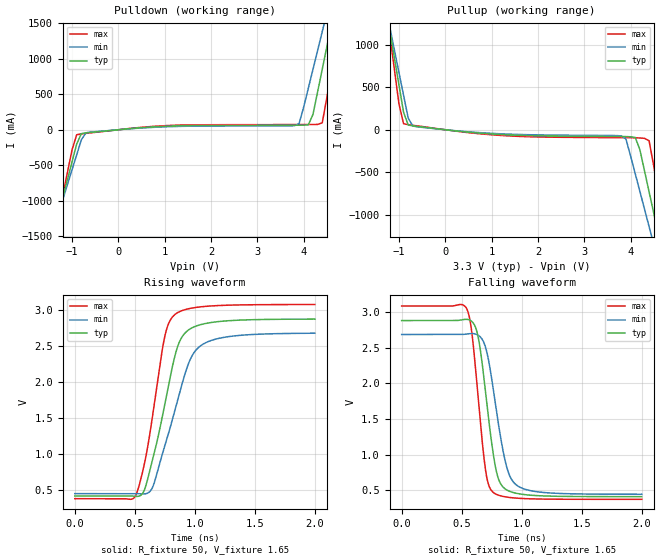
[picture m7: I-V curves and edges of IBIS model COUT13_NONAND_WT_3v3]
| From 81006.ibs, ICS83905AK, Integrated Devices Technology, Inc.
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[Model] COUT13_NONAND_WT_3v3
Model_type   Output
Polarity   Non-Inverting
|   typ   min   max
C_comp   2pF   1.5pF   2.5pF
Vmeas = 1.65V
Rref = 50
Cref = 0
Vref = 1.65V
|   typ   min   max
[Voltage range]   3.3V   3.135V   3.465V
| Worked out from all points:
|   slope of the pulldown table from 0 to 0.495 V, typ, clamps not added: 17.2 ohm
|   slope of the pullup table from 0 to 0.495 V, typ, clamps not added: 17.5 ohm
|   rising waveform, R_fixture 50, V_fixture 1.65: 20-80 % time 191ps typ, 231ps min, 151ps max; typ from 0.413 V to 2.88 V
|   falling waveform, R_fixture 50, V_fixture 1.65: 20-80 % time 111ps typ, 132ps min, 92.3ps max; typ from 2.88 V to 0.413 V
[Pulldown]
|Voltage   I (typ)   I (min)   I (max)
-3.3V     -6.232A    -5.39A     -7.642A
-1.4V     -1.462A    -1.406A    -1.567A
-900mV    -201.6mA   -354.4mA   -70.88mA
-800mV    -55.69mA   -144.2mA   -58.68mA
-600mV    -37.87mA   -33.24mA   -43.91mA
3.9V      63.76mA    86.74mA    73.17mA
4.2V      215.8mA    852.4mA    74.01mA
4.4V      853.2mA    1.385A     97.44mA
4.6V      1.492A     1.918A     860.7mA
4.7V      1.813A     2.186A     1.269A
4.8V      2.133A     2.453A     1.678A
6.6V      8.005A     7.35A      9.166A
[Pullup]
|Voltage   I (typ)   I (min)   I (max)
-3.3V     7.952A     6.873A     9.764A
-1.3V     1.498A     1.483A     1.542A
-1.2V     1.175A     1.214A     1.13A
-900mV    207mA      406.2mA    70.87mA
-700mV    45.36mA    43.45mA    52.59mA
3.8V      -79.66mA   -71.98mA   -93.19mA
4.1V      -90.21mA   -515.7mA   -94.64mA
4.3V      -481.9mA   -931.7mA   -100.8mA
4.4V      -731.3mA   -1.14A     -130mA
4.6V      -1.231A    -1.557A    -746.2mA
4.8V      -1.73A     -1.974A    -1.383A
6.6V      -6.231A    -5.73A     -7.118A
[Ramp]
|   typ   min   max
dV/dt_r   1.976/0.286n   1.791/0.341n   2.171/0.231n
dV/dt_f   1.985/0.169n   1.8/0.205n   2.182/0.138n
R_load =   50.0000
[Rising Waveform]
R_fixture = 50
V_fixture = 1.65   |Vcc_typ
V_fixture_min = 1.5675 |Vcc_min
V_fixture_max = 1.7325 |Vcc_max
C_fixture = 0.0p
| Time   typ   min   max
0s        413mV      446.1mV    375.2mV
504.5ps   407.4mV    446.2mV    411.2mV
574.6ps   477.1mV    441.4mV    819.3mV
646.6ps   907.6mV    529mV      1.514V
750.8ps   1.7V       1.114V     2.643V
834.8ps   2.37V      1.613V     2.943V
886.9ps   2.611V     1.936V     2.992V
959ps     2.74V      2.305V     3.026V
1.079ns   2.813V     2.539V     3.054V
2ns       2.878V     2.681V     3.081V
[Falling Waveform]
R_fixture = 50
V_fixture = 1.65   |Vcc_typ
V_fixture_min = 1.5675 |Vcc_min
V_fixture_max = 1.7325 |Vcc_max
C_fixture = 0.0p
| Time   typ   min   max
0s        2.878V     2.683V     3.082V
542.5ps   2.895V     2.69V      3.042V
584.6ps   2.866V     2.697V     2.71V
638.6ps   2.637V     2.673V     1.766V
702.7ps   1.819V     2.482V     742.2mV
764.8ps   991.3mV    1.9V       469.8mV
808.8ps   650.8mV    1.403V     432mV
868.9ps   513.5mV    867.4mV    408.4mV
963ps     457mV      567.3mV    391.1mV
2ns       413mV      446.3mV    375.2mV
